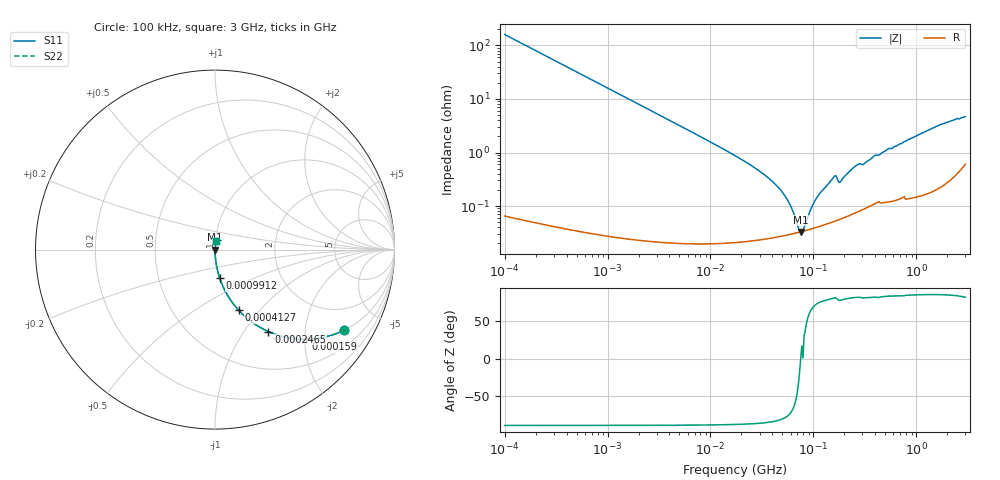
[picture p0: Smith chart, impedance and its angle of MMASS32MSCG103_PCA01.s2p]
! MMASS32MSCG103_PCA01  S-PARAMETER MODEL  ( Standard Model )
! Model Generated by TAIYO YUDEN Corporation (https://www.yuden.co.jp/en/)
! Version 1.0
! TAIYO YUDEN Control No. 250312
! Copyright(c) 2025 TAIYO YUDEN CO.,LTD. All Rights Reserved.
! Product Description (link to TY-COMPAS)
! https://ds.yuden.co.jp/TYCOMPAS/or/detail?pn=MMASS32MSCG103JPCA01&u=M
! Products Name : Multilayer Ceramic Capacitors
! Characteristics :
!  Capacitance : 0.01 [uF] , Rated Voltage : 630 [V] , TCC : CG / C0G
!  Case Size : 3.2 x 2.5 / 0.126 x 0.098 [mm/inch] , Thickness : 2.5 / 0.098 [mm/inch]
!  (Conditions: Temperature = 25 [degC] , DC Bias Voltage = 0 [V])
! External Node Assignments :
!  1  o---| |---o  2
! GND o---------o GND
! Frequency Range : 0.1MHz  -  3000MHz  [ 401 STEP ]
# MHZ S RI R 50
! Freq[MHz].  S11 Real  S11 Imag  S21 Real  S21 Imag  S12 Real  S12 Imag  S22 Real  S22 Imag
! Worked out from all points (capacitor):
!   401 points, 100 kHz to 3 GHz, reference 50 ohm
!   read as one part in series: C = 9.91 nF near 105.3 kHz
!   lowest |Z| = 32.9 mohm at 75.26 MHz (marker M1)
!   series resonance near 75.36 MHz, so ESL is about 450 pH
!   S11 on the Smith chart (normalised r, x): 100 kHz: 1.00, -3.21; 159 kHz: 1.00, -2.02; 246.5 kHz: 1.00, -1.30; 412.7 kHz: 1.00, -0.78; 991.2 kHz: 1.00, -0.32; 3 GHz: 1.01, +0.09
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0.1  0.7205 -0.4485  0.2795 0.4485  0.2795 0.4485  0.7205 -0.4485
0.159027  0.5047 -0.4997  0.4953 0.4997  0.4953 0.4997  0.5047 -0.4997
0.246461  0.298 -0.457  0.702 0.457  0.702 0.457  0.298 -0.457
0.412671  0.1317 -0.3376  0.8683 0.3376  0.8683 0.3376  0.1317 -0.3376
0.562235  0.0756 -0.2638  0.9244 0.2638  0.9244 0.2638  0.0756 -0.2638
0.991196  0.0258 -0.1577  0.9742 0.1577  0.9742 0.1577  0.0258 -0.1577
3.161081  0.00277 -0.0505  0.9972 0.0505  0.9972 0.0505  0.00277 -0.0505
17.7727  0.00028 -0.0085  0.9997 0.0085  0.9997 0.0085  0.00028 -0.0085
32.15051  0.000253 -0.00407  0.9997 0.00407  0.9997 0.00407  0.000253 -0.00407
46.11977  0.000271 -0.00216  0.9997 0.00216  0.9997 0.00216  0.000271 -0.00216
58.15973  0.000293 -0.00111  0.9997 0.00111  0.9997 0.00111  0.000293 -0.00111
71.47675  0.000321 -0.000223  0.9997 0.000223  0.9997 0.000223  0.000321 -0.000223
75.25761  0.000329 -5.52e-06  0.9997 5.52e-06  0.9997 5.52e-06  0.000329 -5.52e-06
81.30716  0.000342 0.000208  0.9997 -0.000208  0.9997 -0.000208  0.000342 0.000208
97.38194  0.000378 0.000922  0.9996 -0.000922  0.9996 -0.000922  0.000378 0.000922
113.6672  0.000415 0.0016  0.9996 -0.0016  0.9996 -0.0016  0.000415 0.0016
158.9065  0.000526 0.00349  0.9995 -0.00349  0.9995 -0.00349  0.000526 0.00349
185.4806  0.000583 0.00287  0.9994 -0.00287  0.9994 -0.00287  0.000583 0.00287
259.3015  0.000781 0.00561  0.9992 -0.00561  0.9992 -0.00561  0.000781 0.00561
547.5153  0.00133 0.0118  0.9987 -0.0118  0.9987 -0.0118  0.00133 0.0118
1658.39  0.00317 0.0321  0.9968 -0.0321  0.9968 -0.0321  0.00317 0.0321
3000  0.0081 0.0457  0.9919 -0.0457  0.9919 -0.0457  0.0081 0.0457
